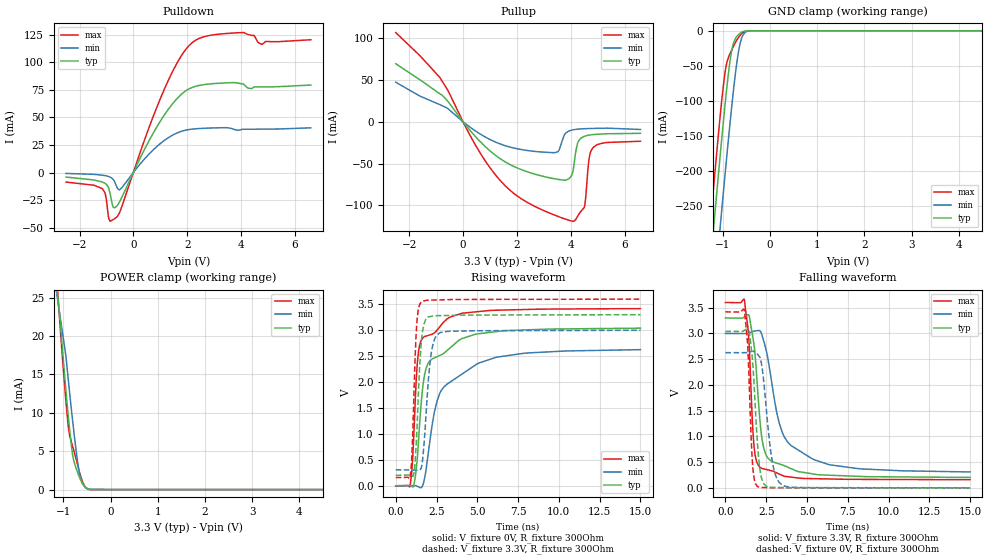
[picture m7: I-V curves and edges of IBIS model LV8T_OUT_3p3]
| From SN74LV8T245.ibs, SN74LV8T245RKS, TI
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[Model]   LV8T_OUT_3p3
Model_type   I/O
Polarity   Non-Inverting
Enable   Active-Low
Vinl = 0.75
Vinh = 1.45
Vmeas = 1.65
Vref = 0
Cref = 2pF
Rref = 100000
|   typ   min   max
C_comp   6.7pF   6.5pF   7pF
[Voltage Range]   3.3   3   3.6
[Temperature Range]   25   125   -40
[Pullup Reference]   3.3   3   3.6
[Pulldown Reference]   0   0   0
[Power Clamp Reference]   3.3   3   3.6
[GND Clamp Reference]   0   0   0
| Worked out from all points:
|   slope of the pulldown table from 0 to 0.495 V, typ, clamps not added: 20 ohm
|   slope of the pullup table from 0 to 0.495 V, typ, clamps not added: 26.2 ohm
|   GND clamp passes 1 mA (typ) near -0.56 V on its own axis
|   POWER clamp passes 1 mA (typ) near -0.61 V on its own axis
|   falling waveform, V_fixture 3.3V, R_fixture 300Ohm: 20-80 % time 528ps typ, 1.31ns min, 311ps max; typ from 3.3 V to 0.203 V
|   rising waveform, V_fixture 0V, R_fixture 300Ohm: 20-80 % time 834ps typ, 1.86ns min, 423ps max; typ from 0 V to 3.04 V
|   rising waveform, V_fixture 3.3V, R_fixture 300Ohm: 20-80 % time 288ps typ, 390ps min, 225ps max; typ from 0.203 V to 3.3 V
|   falling waveform, V_fixture 0V, R_fixture 300Ohm: 20-80 % time 359ps typ, 530ps min, 252ps max; typ from 3.04 V to 0 V
[Pulldown]
|   Voltage   I(typ)   I(min)   I(max)
-2.5V     -4.103mA   -818.3uA   -8.642mA
-1.156V   -8.529mA   -2.393mA   -14.55mA
-1.04V    -9.997mA   -2.857mA   -19.71mA
-862mV    -19.16mA   -4.147mA   -44.16mA
-746.5mV  -31.3mA    -6.307mA   -42.54mA
-589mV    -29.58mA   -14.36mA   -39.56mA
1.165V    52.63mA    29.32mA    76.22mA
1.774V    70.64mA    37.25mA    105.4mA
2.341V    78.3mA     39.68mA    120.2mA
4.062V    80.29mA    39.2mA     126.8mA
4.777V    77.55mA    39.33mA    116.2mA
6.593V    79.24mA    40.5mA     120.3mA
[GND Clamp]
|   Voltage   I(typ)   I(min)   I(max)
-2.5V     -1.32A     -1.415A    -1.27A
-1.292V   -360.1mA   -463.1mA   -301.8mA
-1.24V    -319.7mA   -422.9mA   -261.3mA
-1.198V   -287.6mA   -390.9mA   -229.2mA
-1.145V   -247.9mA   -351.1mA   -189.8mA
-1.051V   -177.9mA   -280.5mA   -121.5mA
-935.5mV  -97.11mA   -196.4mA   -54.1mA
-809.5mV  -29.07mA   -110mA     -27.75mA
-694mV    -7.468mA   -43.15mA   -12.67mA
-578.5mV  -1.458mA   -7.356mA   -2.841mA
-421mV    -17.94uA   -161.4uA   -14.88uA
7.979V    0A         0A         0A
[Pullup]
|   Voltage   I(typ)   I(min)   I(max)
-2.5V     69.3mA     47.24mA    106.5mA
-862mV    33.38mA    20.44mA    52.98mA
1.312V    -42.55mA   -25.66mA   -67.53mA
3.075V    -65.96mA   -36.47mA   -107.2mA
3.517V    -68.74mA   -36.01mA   -112.9mA
3.811V    -69.79mA   -13.65mA   -116.3mA
4.115V    -52.96mA   -9.475mA   -118.8mA
4.262V    -25.19mA   -8.872mA   -112.6mA
4.503V    -17.46mA   -8.338mA   -102.4mA
4.682V    -15.98mA   -8.108mA   -44.46mA
4.84V     -15.31mA   -7.966mA   -30.6mA
6.593V    -13.81mA   -9.25mA    -23.3mA
[POWER Clamp]
|   Voltage   I(typ)   I(min)   I(max)
-2.5V     106.2mA    85.74mA    131.2mA
-1.167V   27.82mA    26.66mA    30.13mA
-1.093V   23.81mA    23.58mA    23.51mA
-946mV    13.06mA    17.45mA    11.64mA
-904mV    10.2mA     14.92mA    8.792mA
-872.5mV  8.231mA    13.02mA    7.316mA
-799mV    4.394mA    8.801mA    5.562mA
-715mV    2.55mA     4.464mA    3.661mA
-652mV    1.525mA    1.908mA    2.177mA
-589mV    715.9uA    794.9uA    961.3uA
-484mV    74.52uA    145.8uA    53.97uA
7.979V    0A         0A         0A
[Ramp]
R_load = 300
|   typ   min   max
dV/dt_r   1.82373/8.29516e-10   1.57531/1.88165e-09   2.05033/4.18727e-10
dV/dt_f   1.85828/5.2601e-10   1.61431/1.30026e-09   2.06483/3.10998e-10
[Falling Waveform]
V_fixture = 3.3V
V_fixture_min = 3V
V_fixture_max = 3.6V
R_fixture = 300Ohm
C_fixture = 0F
|   Time   V(typ)   V(min)   V(max)
0s        3.3V       2.999V     3.6V
1.165ns   3.321V     2.996V     3.646V
1.436ns   3.354V     3.007V     2.894V
1.746ns   2.789V     3.043V     835.2mV
2.144ns   1.216V     3.043V     395.5mV
2.595ns   581.7mV    2.527V     349.9mV
3.302ns   464.1mV    1.254V     268.3mV
4.012ns   375.1mV    823.9mV    209.4mV
6.373ns   245.5mV    448.8mV    172.8mV
15ns      202.5mV    308.8mV    158.4mV
[Rising Waveform]
V_fixture = 0V
V_fixture_min = 0V
V_fixture_max = 0V
R_fixture = 300Ohm
C_fixture = 0F
|   Time   V(typ)   V(min)   V(max)
0s        71.13uV    163.1uV    37.48uV
886.8ps   4.43mV     2.171mV    8.603mV
1.04ns    -23.36mV   2.518mV    537.5mV
1.209ns   186.5mV    2.901mV    1.731V
1.505ns   1.37V      -36.76mV   2.758V
1.927ns   2.324V     469.6mV    2.893V
2.527ns   2.489V     1.63V      2.999V
3.16ns    2.613V     1.963V     3.221V
6.151ns   2.973V     2.479V     3.386V
15ns      3.04V      2.626V     3.417V
[Rising Waveform]
V_fixture = 3.3V
V_fixture_min = 3V
V_fixture_max = 3.6V
R_fixture = 300Ohm
C_fixture = 0F
|   Time   V(typ)   V(min)   V(max)
0s        202.5mV    308.8mV    158.4mV
890.5ps   205.9mV    304.3mV    180.3mV
982.3ps   192mV      303.9mV    542.7mV
1.118ns   253.2mV    303.2mV    1.781V
1.276ns   930.2mV    302.4mV    3.062V
1.46ns    2.264V     303.2mV    3.488V
1.594ns   2.854V     385.2mV    3.555V
2.144ns   3.266V     2.485V     3.581V
2.672ns   3.281V     2.946V     3.585V
15ns      3.3V       2.999V     3.6V
[Falling Waveform]
|Gnd
V_fixture = 0V
V_fixture_min = 0V
V_fixture_max = 0V
R_fixture = 300Ohm
C_fixture = 0F
|   Time   V(typ)   V(min)   V(max)
0s        3.04V      2.626V     3.417V
1.165ns   3.059V     2.626V     3.442V
1.38ns    3.072V     2.632V     2.681V
1.665ns   2.459V     2.653V     461.6mV
1.946ns   950.6mV    2.603V     29.39mV
2.147ns   297.4mV    2.504V     10.79mV
2.351ns   82.12mV    2.062V     6.346mV
2.902ns   8.065mV    459.9mV    3.079mV
3.498ns   4.496mV    53.95mV    2.93mV
15ns      71.4uV     163.9uV    37.52uV
